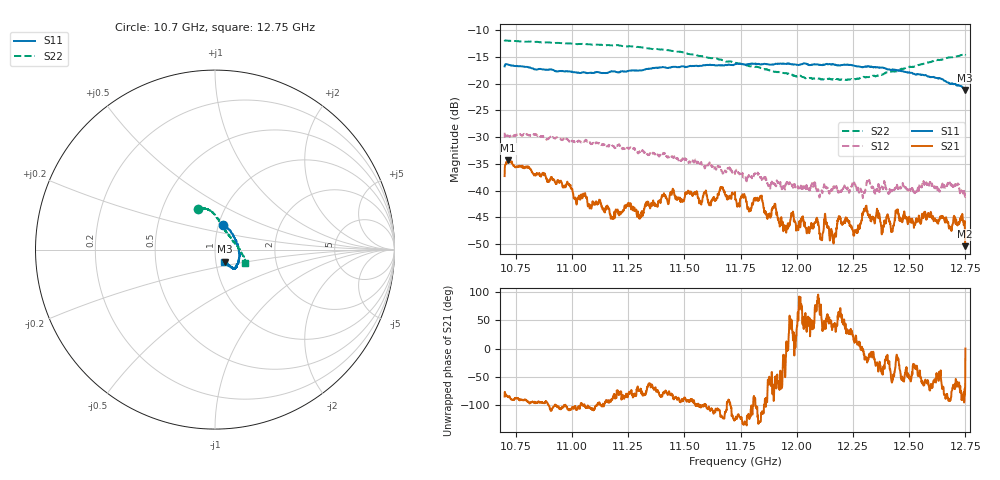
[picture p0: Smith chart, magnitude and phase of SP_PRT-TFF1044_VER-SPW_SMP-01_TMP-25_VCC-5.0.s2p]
!Agilent Technologies,N5230A,US43500178,A.04.87.01
!Agilent N5230A: A.04.87.01
!Date: Tuesday, January 13, 2015 19:26:56
!Correction: S11(Full 2 Port TRL,1,2) S21(Full 2 Port TRL,1,2) S12(Full 2 Port TRL,1,2) S22(Full 2 Port TRL,1,2)
!S2P File: Measurements: S11, S21, S12, S22:
# Hz S  dB  R 50
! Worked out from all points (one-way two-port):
!   2051 points, 10.7 GHz to 12.75 GHz, reference 50 ohm
!   highest |S21| = -34.36 dB at 10.72 GHz (marker M1); lowest = -50.4 dB at 12.75 GHz (marker M2)
!   lowest |S11| = -21.2 dB at 12.75 GHz (marker M3), VSWR 1.19, Z = 55.3 - j7.59 ohm
!   |S11| at or under -10 dB: start of sweep to end of sweep
!   |S22| runs from -19.3 to -11.9 dB; largest |S21 - S12| = 0.029
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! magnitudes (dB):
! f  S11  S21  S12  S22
! 10.7 GHz  -16.8  -37.3  -29.2  -12.1
! 10.72 GHz  -16.4  -34.4  -29.7  -12.0
! 11.04 GHz  -18.0  -40.9  -31.0  -12.6
! 11.18 GHz  -17.7  -45.3  -31.7  -12.8
! 11.38 GHz  -17.0  -42.1  -33.4  -13.6
! 11.45 GHz  -16.9  -40.4  -33.6  -13.9
! 11.72 GHz  -16.4  -40.3  -36.9  -16.1
! 11.79 GHz  -16.3  -43.5  -37.7  -16.7
! 11.84 GHz  -16.4  -41.0  -37.5  -17.1
! 11.95 GHz  -16.3  -47.0  -38.8  -18.0
! 11.98 GHz  -16.4  -44.6  -39.1  -18.4
! 12.07 GHz  -16.4  -46.4  -38.6  -19.1
! 12.11 GHz  -16.5  -49.1  -39.9  -19.2
! 12.13 GHz  -16.3  -46.4  -39.5  -19.1
! 12.16 GHz  -16.4  -49.1  -39.4  -19.2
! 12.22 GHz  -16.4  -45.4  -39.8  -19.3
! 12.26 GHz  -16.7  -47.5  -39.5  -19.2
! 12.3 GHz  -16.8  -43.8  -40.0  -18.8
! 12.41 GHz  -17.3  -45.3  -40.3  -17.8
! 12.74 GHz  -20.7  -44.3  -40.2  -14.6
! 12.75 GHz  -21.2  -50.4  -41.2  -14.6
! 12.75 GHz  -21.1  -49.9  -41.1  -14.7
